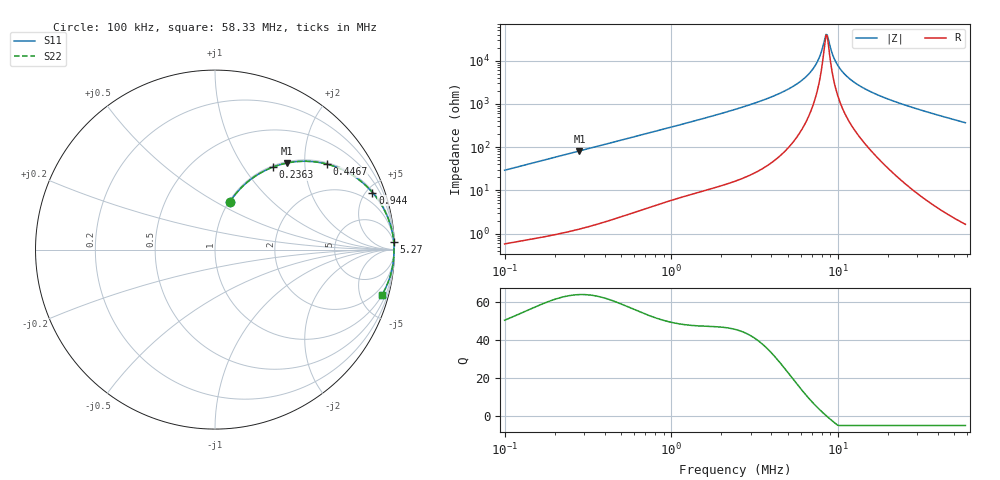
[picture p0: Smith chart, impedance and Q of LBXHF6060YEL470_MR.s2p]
! LBXHF6060YEL470_MR  S-PARAMETER MODEL  ( General Type )
! Model Generated by TAIYO YUDEN Corporation (http://www.ty-top.com)
! Version 1.0
! TAIYO YUDEN Control No. 200120NI43SB-FBB
! Copyright(c) 2020 TAIYO YUDEN CO.,LTD. All Rights Reserved.
! Product Description (link to TY-COMPAS)
! https://ds.yuden.co.jp/TYCOMPAS/or/detail?pn=LBXHF6060YEL470MMR&u=M
! Products Name : Inductors
! Characteristics :
!  Inductance : 47 uH , SRF(min) : 6.0 MHz , DC Resistance(max) : 0.272 Ohm
!  Rated Current : Saturation :1550 mA , Temp Rise : 700 mA
!  Case Size : 6.0 x 6.0 / 0.236 x 0.236 [mm/inch] , Thickness : 4.5 / 0.177 [mm/inch]
!  (Conditions: Temperature = 25 degC , DC Bias Current/Voltage = 0A / 0V)
! External Node Assignments :
!  1  o---GGG---o  2
! GND o---------o GND
! Frequency Range : 0.1MHz  -  58.334721MHz  [ 402 STEP ]
# MHz S RI R 50
! Freq[MHz].  S11 Real  S11 Imag  S21 Real  S21 Imag  S12 Real  S12 Imag  S22 Real  S22 Imag
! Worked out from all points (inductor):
!   401 points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, 100 kHz to 58.33 MHz, reference 50 ohm
!   read as one part in series: L = 46.3 uH near 103.2 kHz
!   highest Q = 64.1 at 281.5 kHz (marker M1), where L = 46.1 uH
!   self-resonance near 8.496 MHz
!   S11 on the Smith chart (normalised r, x): 100 kHz: 1.01, +0.58; 236.3 kHz: 1.02, +1.37; 446.7 kHz: 1.04, +2.59; 944 kHz: 1.11, +5.47; 5.27 MHz: 3, +48; 58.33 MHz: 1.03, -7.33
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0.1  0.083 0.2662  0.917 -0.2662  0.917 -0.2662  0.083 0.2662
0.156176  0.1753 0.3717  0.8247 -0.3717  0.8247 -0.3717  0.1753 0.3717
0.236265  0.3224 0.4595  0.6776 -0.4595  0.6776 -0.4595  0.3224 0.4595
0.28149  0.4014 0.4824  0.5986 -0.4824  0.5986 -0.4824  0.4014 0.4824
0.290598  0.4165 0.4852  0.5835 -0.4852  0.5835 -0.4852  0.4165 0.4852
0.446676  0.6239 0.4762  0.3761 -0.4762  0.3761 -0.4762  0.6239 0.4762
0.844473  0.852 0.3454  0.148 -0.3454  0.148 -0.3454  0.852 0.3454
0.944038  0.8774 0.3181  0.1226 -0.3181  0.1226 -0.3181  0.8774 0.3181
2.454022  0.9801 0.129  0.0199 -0.129  0.0199 -0.129  0.9801 0.129
3.832598  0.9925 0.0729  0.00745 -0.0729  0.00745 -0.0729  0.9925 0.0729
5.269745  0.9963 0.0412  0.00371 -0.0412  0.00371 -0.0412  0.9963 0.0412
6.179279  0.9972 0.027  0.00283 -0.027  0.00283 -0.027  0.9972 0.027
7.018695  0.9975 0.0162  0.00247 -0.0162  0.00247 -0.0162  0.9975 0.0162
7.722275  0.9976 0.00833  0.00238 -0.00833  0.00238 -0.00833  0.9976 0.00833
8.362177  0.9976 0.00186  0.0024 -0.00186  0.0024 -0.00186  0.9976 0.00186
8.632746  0.9976 -0.000712  0.00243 0.000712  0.00243 0.000712  0.9976 -0.000712
9.650564  0.9974 -0.0097  0.00262 0.0097  0.00262 0.0097  0.9974 -0.0097
10.28518  0.9972 -0.0149  0.00278 0.0149  0.00278 0.0149  0.9972 -0.0149
11.13746  0.997 -0.0214  0.00304 0.0214  0.00304 0.0214  0.997 -0.0214
14.14192  0.9958 -0.0419  0.00421 0.0419  0.00421 0.0419  0.9958 -0.0419
20.39619  0.9918 -0.0787  0.00815 0.0787  0.00815 0.0787  0.9918 -0.0787
58.33472  0.9297 -0.2534  0.0703 0.2534  0.0703 0.2534  0.9297 -0.2534
